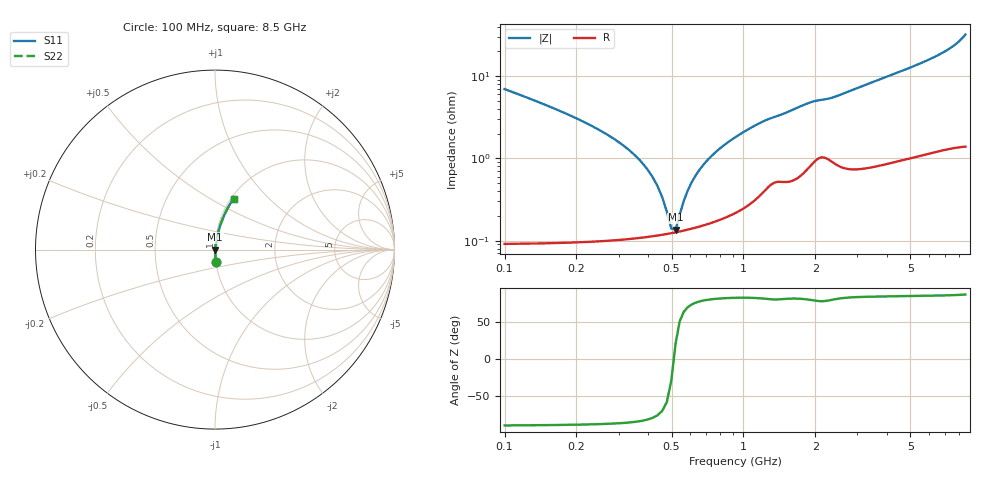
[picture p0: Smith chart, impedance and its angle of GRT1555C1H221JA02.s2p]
!Murata Part Number: GRT1555C1H221JA02
!These Parameters are Measured in Series Mode Connection
!Data Generated on Jun 19, 2026
!  o--ll--o
!Port1  Port2
!  o------o
!Operation Temp=25[degC], DC Bias Voltage=0[V]
!Freq. Start=100[MHz] Stop=9[GHz] 401[Steps]
# Hz S RI R 50
!Freq.(Hz) S11(Real) S11(Imag) S21(Real) S21(Imag) S12(Real) S12(Imag) S22(Real) S22(Imag)
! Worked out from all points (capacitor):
!   401 points, 100 MHz to 8.5 GHz, reference 50 ohm
!   read as one part in series: C = 220 pF near 142 MHz
!   lowest |Z| = 136 mohm at 520 MHz (marker M1)
!   series resonance near 511 MHz, so ESL is about 440 pH
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1e8  0.00572 -0.0691  0.9943 0.0691  0.9943 0.0691  0.00572 -0.0691
1.42e8  0.00313 -0.0468  0.9969 0.0468  0.9969 0.0468  0.00313 -0.0468
3.52e8  0.00118 -0.0108  0.9988 0.0108  0.9988 0.0108  0.00118 -0.0108
4.15e8  0.00116 -0.00592  0.9988 0.00592  0.9988 0.00592  0.00116 -0.00592
4.78e8  0.00121 -0.00189  0.9988 0.00189  0.9988 0.00189  0.00121 -0.00189
4.99e8  0.00123 -0.000669  0.9988 0.000669  0.9988 0.000669  0.00123 -0.000669
5.2e8  0.00126 0.000497  0.9987 -0.000497  0.9987 -0.000497  0.00126 0.000497
5.41e8  0.00129 0.00162  0.9987 -0.00162  0.9987 -0.00162  0.00129 0.00162
6.04e8  0.00141 0.00476  0.9986 -0.00476  0.9986 -0.00476  0.00141 0.00476
6.46e8  0.00151 0.0067  0.9985 -0.0067  0.9985 -0.0067  0.00151 0.0067
7.09e8  0.00168 0.00945  0.9983 -0.00945  0.9983 -0.00945  0.00168 0.00945
8.14e8  0.00202 0.0137  0.998 -0.0137  0.998 -0.0137  0.00202 0.0137
9.61e8  0.00266 0.0192  0.9973 -0.0192  0.9973 -0.0192  0.00266 0.0192
1.129e9  0.00381 0.0251  0.9962 -0.0251  0.9962 -0.0251  0.00381 0.0251
1.276e9  0.00539 0.0295  0.9946 -0.0295  0.9946 -0.0295  0.00539 0.0295
1.507e9  0.00637 0.0351  0.9936 -0.0351  0.9936 -0.0351  0.00637 0.0351
1.927e9  0.0105 0.0468  0.9895 -0.0468  0.9895 -0.0468  0.0105 0.0468
2.914e9  0.0119 0.0676  0.9881 -0.0676  0.9881 -0.0676  0.0119 0.0676
4.3e9  0.0199 0.1036  0.9801 -0.1036  0.9801 -0.1036  0.0199 0.1036
5.707e9  0.0319 0.1427  0.9681 -0.1427  0.9681 -0.1427  0.0319 0.1427
7.114e9  0.0519 0.1928  0.9481 -0.1928  0.9481 -0.1928  0.0519 0.1928
8.5e9  0.1032 0.2834  0.8968 -0.2834  0.8968 -0.2834  0.1032 0.2834
